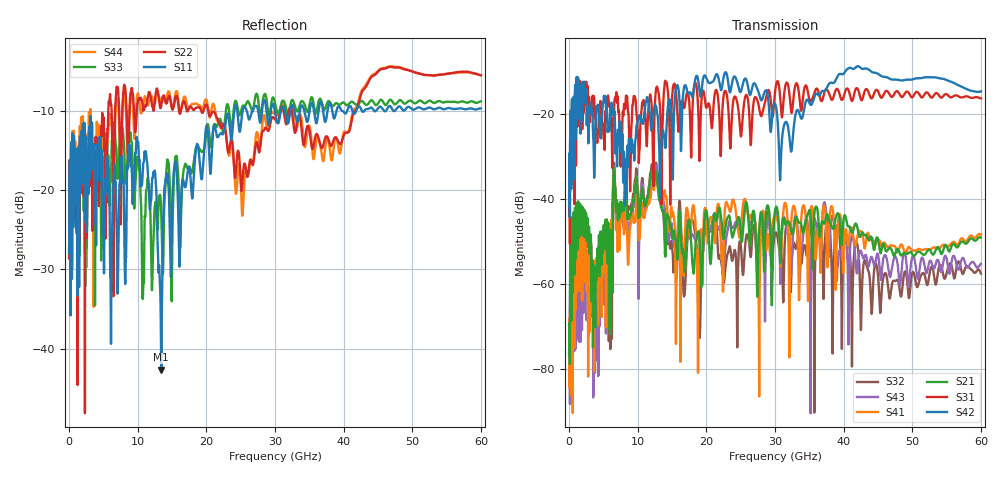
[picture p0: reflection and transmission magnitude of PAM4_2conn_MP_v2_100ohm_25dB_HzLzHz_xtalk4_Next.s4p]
! Info: Touchstone file created by Circ.  Input file=FAB50GbE_2conn_Midplane_Examax_Topo2_v2_100ohm_25dB_HzLzHz.circ
# Hz S RI R 50
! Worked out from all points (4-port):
!   6000 points, 10 MHz to 60 GHz, reference 50 ohm
!   strongest paths, dB at 10 MHz, 15.01 GHz, 30.01 GHz, 45.01 GHz, 60 GHz:
!     S42: -41.6, -24.7, -17.5, -10.5, -14.7
!     S31: -43.9, -16.2, -14.8, -14.6, -16.3
!     S21: -76.2, -49.2, -42.7, -49.5, -49.1
!     S41: -68.2, -44.0, -44.0, -49.6, -48.3
!     S43: -71.3, -47.4, -43.5, -53.0, -55.2
!     S32: -75.3, -51.2, -48.2, -57.9, -57.5
!   lowest |S11| = -42.7 dB at 13.44 GHz (marker M1), VSWR 1.01, Z = 49.4 - j0.413 ohm
!   |S11| at or under -10 dB: start of sweep to 24.09 GHz; 25.88 GHz to 26.75 GHz (875.3 MHz wide, 3.33 % of centre); 29.97 GHz to 30.86 GHz (894.6 MHz wide, 2.94 % of centre)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
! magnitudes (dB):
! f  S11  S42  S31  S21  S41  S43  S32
! 10 MHz  -28.0  -41.6  -43.9  -76.2  -68.2  -71.3  -75.3
! 1.33 GHz  -15.8  -11.4  -12.1  -40.6  -48.8  -54.3  -48.7
! 3.56 GHz  -14.3  -26.4  -18.1  -56.0  -55.3  -68.0  -64.1
! 13.44 GHz  -42.7  -27.8  -29.7  -41.7  -39.5  -40.5  -41.2
! 19 GHz  -16.2  -14.4  -30.9  -49.5  -50.8  -58.4  -72.2
! 21.18 GHz  -11.8  -11.7  -15.8  -43.3  -49.1  -43.4  -44.0
! 60 GHz  -9.7  -14.7  -16.3  -49.1  -48.3  -55.2  -57.5
